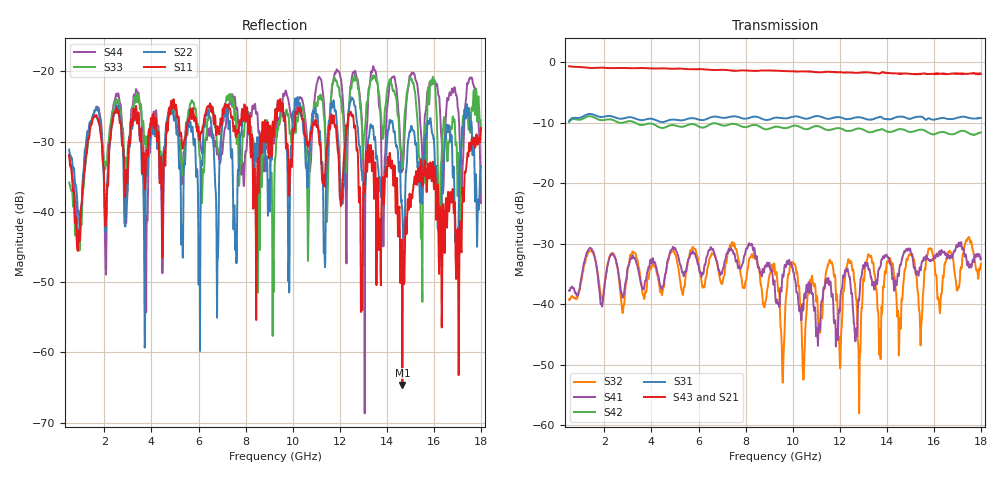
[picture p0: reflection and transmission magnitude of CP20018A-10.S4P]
! Amtery
! Email: info@amtery.com
! Phone: 886-2-2883-7839
! Model Number: CP20018A-10
! 4-port S-parameter measurement data for Bi-Directional Coupler
! Frequency Range: 0.5 GHz to 18 GHz
! Port 1: Input
! Port 2: Output
! Port 3: Coupled Forward
! Port 4: Coupled Reverse
# Hz S dB R 50
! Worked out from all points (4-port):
!   1401 points, 500 MHz to 18 GHz, reference 50 ohm
!   strongest paths, dB at 500 MHz, 4.875 GHz, 9.25 GHz, 13.62 GHz, 18 GHz:
!     S43: -0.6, -1.0, -1.4, -1.8, -1.9
!     S21: -0.6, -1.1, -1.5, -1.7, -2.0
!     S31: -9.7, -9.5, -9.1, -9.1, -9.2
!     S42: -9.9, -10.4, -10.6, -11.2, -11.6
!     S41: -37.7, -30.9, -37.9, -35.2, -32.5
!     S32: -39.3, -31.1, -34.8, -41.0, -33.3
!   lowest |S11| = -64.7 dB at 14.66 GHz (marker M1), VSWR 1.00, Z = 50 + j0.0496 ohm
!   |S11| at or under -10 dB: start of sweep to end of sweep
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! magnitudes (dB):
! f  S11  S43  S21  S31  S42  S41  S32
! 500 MHz  -31.9  -0.6  -0.6  -9.7  -9.9  -37.7  -39.3
! 7.562 GHz  -28.6  -1.4  -1.4  -8.9  -10.2  -32.5  -30.8
! 10.18 GHz  -26.1  -1.5  -1.6  -8.9  -10.5  -38.1  -34.8
! 11.38 GHz  -35.0  -1.5  -1.6  -9.2  -11.0  -37.0  -36.4
! 12.47 GHz  -25.8  -1.6  -1.7  -9.3  -11.3  -37.5  -32.9
! 14.66 GHz  -64.7  -1.8  -1.8  -9.0  -11.1  -32.4  -39.0
! 18 GHz  -28.1  -1.9  -2.0  -9.2  -11.6  -32.5  -33.3
